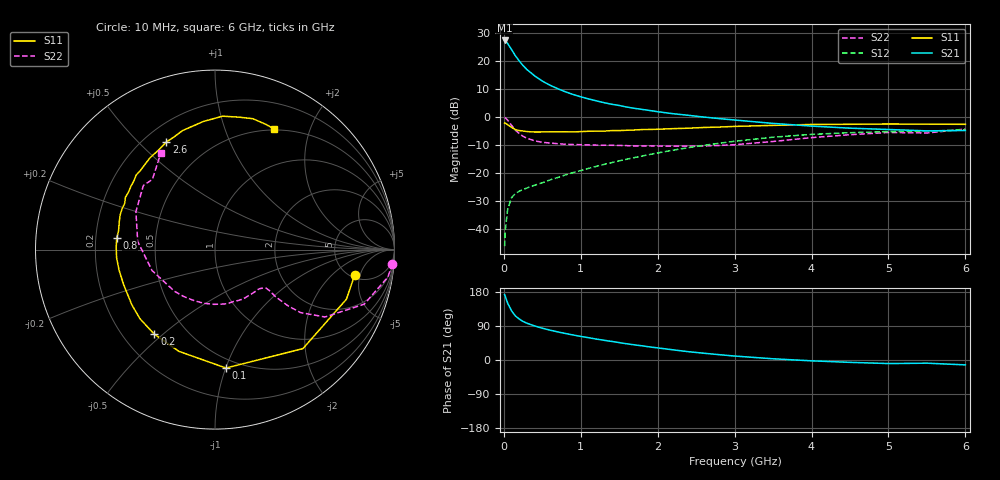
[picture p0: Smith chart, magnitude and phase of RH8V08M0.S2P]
! SIEMENS Small Signal Semiconductors
! BFR106
! Si NPN RF Bipolar Junction Transistor in SOT23
! VCE = 8 V  IC = 8 mA
! Common Emitter S-Parameters:  August  1996
# GHz  S  MA  R  50
!  f  S11  S21  S12  S22
! GHz  MAG  ANG  MAG  ANG  MAG  ANG  MAG  ANG
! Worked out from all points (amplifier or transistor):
!   36 points, 10 MHz to 6 GHz, reference 50 ohm
!   highest |S21| = 27.4 dB at 10 MHz (marker M1)
!   |S21| within 3 dB of that: start of sweep to 94.54 MHz
!   unconditionally stable (mu >= 1): 531.2 MHz to 1.921 GHz; 5.247 GHz to end of sweep
!   at 250 MHz: K = 0.63, MSG = 22.1 dB, |S12| = -25.8 dB
!   at 1.4 GHz: K = 1.10, MAG = 8.6 dB, |S12| = -16.2 dB
!   at 6 GHz: K = 1.01, MAG = -0.8 dB, |S12| = -4.4 dB
!   S11 on the Smith chart (normalised r, x): 10 MHz: 5.33, -4.10; 100 MHz: 0.43, -1.00; 200 MHz: 0.33, -0.47; 800 MHz: 0.29, +0.05; 2.6 GHz: 0.29, +0.61; 6 GHz: 0.48, +1.49
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0.01  0.7907 -10.5  23.52 172.7  0.005 87.9  0.9903 -4.5
0.02  0.7826 -20.7  23.23 167.0  0.01 78.5  0.9758 -9.0
0.05  0.7377 -48.4  20.7 149.7  0.0229 67.0  0.8852 -20.1
0.1  0.6626 -84.7  16.21 129.9  0.0366 55.1  0.7186 -31.5
0.15  0.6015 -109.5  12.54 116.3  0.0435 47.3  0.591 -36.4
0.2  0.58 -125.6  10.15 108.2  0.0479 46.0  0.5123 -37.6
0.25  0.5685 -137.4  8.366 101.6  0.0515 45.4  0.4565 -37.8
0.3  0.5561 -146.4  7.113 97.1  0.0546 46.5  0.4236 -37.8
0.4  0.5452 -159.1  5.493 89.9  0.0612 49.3  0.3797 -37.0
0.5  0.5467 -168.0  4.426 83.9  0.0678 52.0  0.3575 -37.0
0.6  0.5502 -175.4  3.737 78.8  0.0761 54.6  0.3466 -38.0
0.8  0.5512 173.3  2.849 70.0  0.0935 58.8  0.3298 -41.4
0.9  0.5472 169.1  2.551 66.0  0.103 60.6  0.3262 -43.2
1.1  0.5627 159.9  2.129 58.8  0.1221 62.4  0.3213 -49.0
1.3  0.5653 152.8  1.825 52.1  0.1438 63.4  0.3169 -55.0
1.6  0.5866 143.0  1.521 42.7  0.1789 63.5  0.3115 -65.7
2.2  0.627 125.2  1.158 26.8  0.2588 59.4  0.3051 -91.2
2.6  0.6578 114.3  1.009 17.9  0.3154 54.5  0.3072 -112.0
3.5  0.7167 95.2  0.777 3.2  0.441 40.0  0.3696 -161.6
4.5  0.7499 79.8  0.639 -6.2  0.531 21.3  0.4886 154.4
5.5  0.7531 67.9  0.572 -8.4  0.5637 8.8  0.5243 131.7
6  0.7488 64.1  0.58 -12.9  0.5995 0.7  0.6164 119.3
